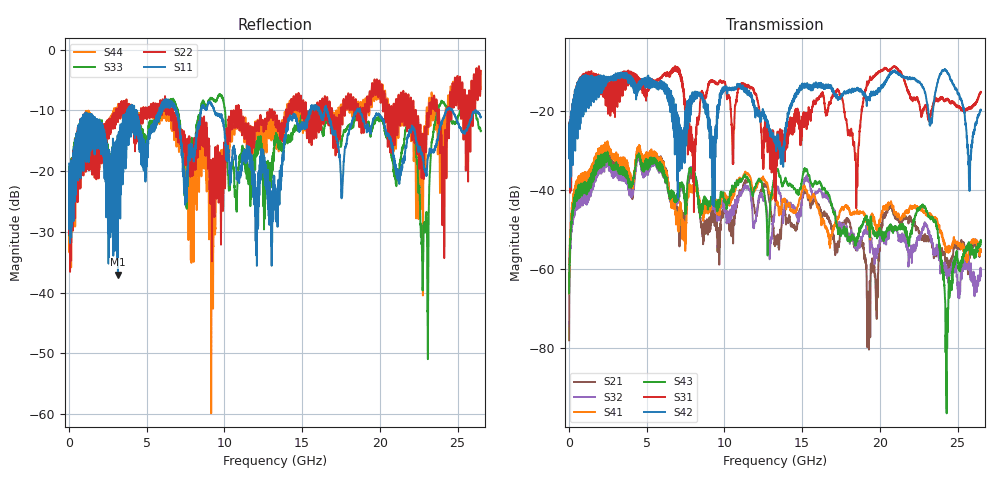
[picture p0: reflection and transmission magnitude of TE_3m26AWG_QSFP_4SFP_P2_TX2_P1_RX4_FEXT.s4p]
!Agilent Technologies,N5222A,MY51421691,A.10.00.00
!Agilent N5222A: A.10.00.00
!Date: Friday, January 30, 2015 12:37:13
!Correction: S11(Full 4 Port(1,2,3,4))
!S12(Full 4 Port(1,2,3,4))
!S13(Full 4 Port(1,2,3,4))
!S14(Full 4 Port(1,2,3,4))
!S21(Full 4 Port(1,2,3,4))
!S22(Full 4 Port(1,2,3,4))
!S23(Full 4 Port(1,2,3,4))
!S24(Full 4 Port(1,2,3,4))
!S31(Full 4 Port(1,2,3,4))
!S32(Full 4 Port(1,2,3,4))
!S33(Full 4 Port(1,2,3,4))
!S34(Full 4 Port(1,2,3,4))
!S41(Full 4 Port(1,2,3,4))
!S42(Full 4 Port(1,2,3,4))
!S43(Full 4 Port(1,2,3,4))
!S44(Full 4 Port(1,2,3,4))
!S4P File: Measurements: <S11,S12,S13,S14>,
!<S21,S22,S23,S24>,
!<S31,S32,S33,S34>,
!<S41,S42,S43,S44>:
# Hz S  dB  R 50.0
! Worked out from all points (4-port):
!   2650 points, 10 MHz to 26.5 GHz, reference 50 ohm
!   strongest paths, dB at 10 MHz, 6.63 GHz, 13.26 GHz, 19.88 GHz, 26.5 GHz:
!     S42: -25.0, -19.4, -27.0, -15.1, -19.8
!     S31: -24.9, -10.2, -30.2, -10.6, -15.3
!     S43: -66.1, -40.4, -36.7, -51.0, -53.2
!     S41: -66.2, -42.7, -42.3, -49.9, -55.7
!     S32: -59.6, -41.6, -44.5, -54.1, -60.7
!     S21: -78.0, -41.6, -54.0, -61.2, -55.3
!   lowest |S11| = -37.1 dB at 3.15 GHz (marker M1), VSWR 1.03, Z = 50.6 - j1.28 ohm
!   |S11| at or under -10 dB: start of sweep to 3.77 GHz; 9.35 GHz to 15.5 GHz (6.146 GHz wide, 49.5 % of centre); 18.72 GHz to 24.29 GHz (5.566 GHz wide, 25.9 % of centre)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
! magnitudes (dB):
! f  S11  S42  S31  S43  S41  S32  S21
! 10 MHz  -18.8  -25.0  -24.9  -66.1  -66.2  -59.6  -78.0
! 3.15 GHz  -37.1  -11.8  -16.9  -33.7  -31.1  -35.2  -33.0
! 18.5 GHz  -10.2  -14.6  -39.2  -52.0  -45.8  -53.4  -53.5
! 19.27 GHz  -12.8  -17.2  -13.1  -48.2  -48.9  -50.3  -69.5
! 22.81 GHz  -18.4  -14.4  -19.7  -44.4  -45.6  -49.2  -52.0
! 24.29 GHz  -10.0  -10.1  -17.1  -95.4  -54.4  -60.6  -57.9
! 26.5 GHz  -11.1  -19.8  -15.3  -53.2  -55.7  -60.7  -55.3
